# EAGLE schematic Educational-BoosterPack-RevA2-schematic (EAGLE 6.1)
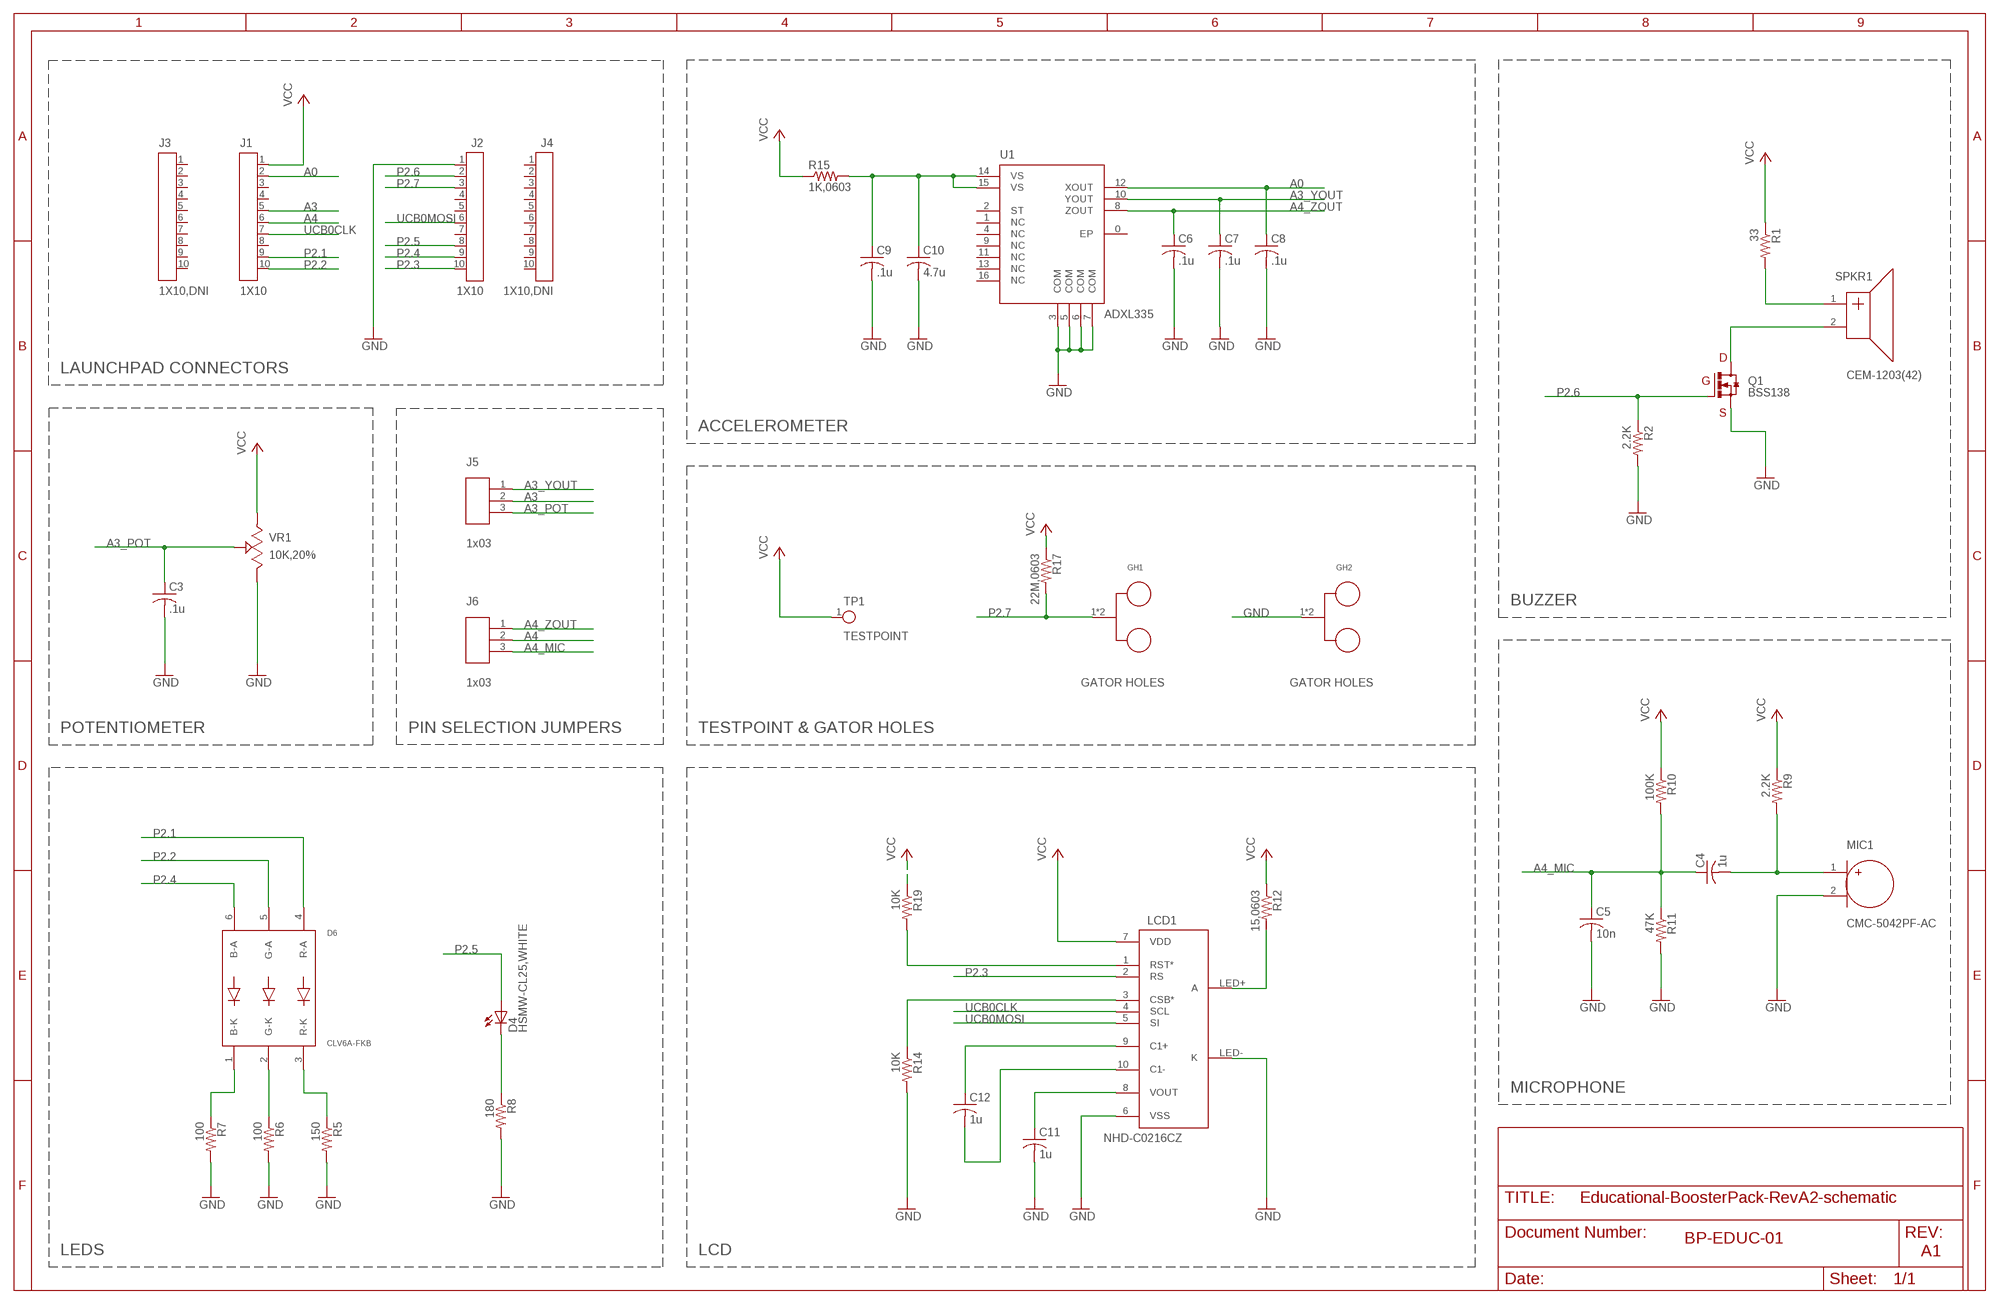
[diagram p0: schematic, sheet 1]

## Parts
C3  .1u  C-USC0402  [C0402]
C4  1u  C-USC0402  [C0402]
C5  10n  C-USC0402  [C0402]
C6  .1u  C-USC0402  [C0402]
C7  .1u  C-USC0402  [C0402]
C8  .1u  C-USC0402  [C0402]
C9  .1u  C-USC0402  [C0402]
C10  4.7u  C-USC0603  [C0603]
C11  1u  C-USC0402  [C0402]
C12  1u  C-USC0402  [C0402]
D4  HSMW-CL25,WHITE  LEDCHIPLED_0603  [CHIPLED_0603]
D6  CLV6A-FKB  [TRICOLOR-LED6]
GH1  MAKEYMAKEY  [MAKEYMAKEY]
GH2  MAKEYMAKEY  [MAKEYMAKEY]
J1  1X10  HEADER1X10  [1X10]
J2  1X10  HEADER1X10  [1X10]
J3  1X10,DNI  HEADER1X10  [1X10]
J4  1X10,DNI  HEADER1X10  [1X10]
J5  1x03  HEADER1X03  [1X03]
J6  1x03  HEADER1X03  [1X03]
LCD1  NHD-C0216CZ  [GENERIC-LCD10-2]
MIC1  CMC-5042PF-AC  [GENERIC-2PADS2]
Q1  BSS138  [SOT23-3]
R1  33  R-US_R0402  [R0402]
R2  2.2K  R-US_R0402  [R0402]
R5  150  R-US_R0402  [R0402]
R6  100  R-US_R0402  [R0402]
R7  100  R-US_R0402  [R0402]
R8  180  R-US_R0402  [R0402]
R9  2.2K  R-US_R0402  [R0402]
R10  100K  R-US_R0402  [R0402]
R11  47K  R-US_R0402  [R0402]
R12  15,0603  R-US_R0603  [R0603]
R14  10K  R-US_R0402  [R0402]
R15  1K,0603  R-US_R0603  [R0603]
R17  22M,0603  R-US_R0603  [R0603]
R19  10K  R-US_R0402  [R0402]
SPKR1  CEM-1203(42)  [GENERIC-2PADS]
TP1  TESTPOINT  [TESTPOINT]
U1  ADXL335  [LFCSP-16]
VR1  10K,20%  3352T  [GENERIC-3HOLES]

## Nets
A0: C8.1 J1.2 U1.12(XOUT)
A3: J1.5 J5.2
A3_POT: C3.1 J5.3 VR1.2
A3_YOUT: C7.1 J5.1 U1.10(YOUT)
A4: J1.6 J6.2
A4_MIC: C4.1 C5.1 J6.3 R10.2 R11.1
A4_ZOUT: C6.1 J6.1 U1.8(ZOUT)
GND: C3.2 C5.2 C6.2 C7.2 C8.2 C9.2 C10.2 C11.2 GH2.1 GH2.2 J2.1 LCD1.6(VSS) LCD1.LED-(K) MIC1.2(MIC_N) Q1.2(S) R2.2 R5.2 R6.2 R7.2 R8.2 R11.2 R14.2 U1.3(COM) U1.5(COM) U1.6(COM) U1.7(COM) VR1.3
N$1: C9.1 C10.1 R15.2 U1.14(VS) U1.15(VS)
N$2: C4.2 MIC1.1(MIC_P) R9.2
N$3: LCD1.LED+(A) R12.2
N$4: D6.2(G-K) R6.1
N$5: R1.2 SPKR1.1(SPKR_P)
N$6: Q1.3(D) SPKR1.2(SPKR_N)
N$7: LCD1.3(CSB*) R14.1
N$8: D6.3(R-K) R5.1
N$9: D6.1(B-K) R7.1
N$10: C11.1 LCD1.8(VOUT)
N$11: C12.2 LCD1.10(C1-)
N$12: C12.1 LCD1.9(C1+)
N$13: LCD1.1(RST*) R19.2
N$16: D4.C R8.1
P2.1: D6.4(R-A) J1.9
P2.2: D6.5(G-A) J1.10
P2.3: J2.10 LCD1.2(RS)
P2.4: D6.6(B-A) J2.9
P2.5: D4.A J2.8
P2.6: J2.2 Q1.1(G) R2.1
P2.7: GH1.1 GH1.2 J2.3 R17.2
UCB0CLK: J1.7 LCD1.4(SCL)
UCB0MOSI: J2.6 LCD1.5(SI)
VCC: J1.1 LCD1.7(VDD) R1.1 R9.1 R10.1 R12.1 R15.1 R17.1 R19.1 TP1.1 VR1.1
Unconnected: J1.3 J1.4 J1.8 J2.4 J2.5 J2.7 J3.1 J3.2 J3.3 J3.4 J3.5 J3.6 J3.7 J3.8 J3.9 J3.10 J4.1 J4.2 J4.3 J4.4 J4.5 J4.6 J4.7 J4.8 J4.9 J4.10 U1.0(EP) U1.1(NC) U1.2(ST) U1.4(NC) U1.9(NC) U1.11(NC) U1.13(NC) U1.16(NC)

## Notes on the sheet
- LAUNCHPAD CONNECTORS
- ACCELEROMETER
- BUZZER
- GATOR HOLES | GATOR HOLES
- POTENTIOMETER | PIN SELECTION JUMPERS | TESTPOINT & GATOR HOLES
- MICROPHONE
- BP-EDUC-01
- LEDS | LCD | A1

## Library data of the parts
C3-C12 = resistor:C-US: CAPACITOR, American symbol
D4 = led:LED: LED
D6 = CCo-Boost:CLV6A-FKB
GH1 GH2 = CCo-Boost:MAKEYMAKEY
J1-J4 = CCo-Boost:HEADER1X10
J5 J6 = CCo-Boost:HEADER1X03
LCD1 = CCo-Boost:NHD-C0216CZ
MIC1 = CCo-Boost:CMC-5042PF-AC
Q1 = CCo-Boost:BSS138: BSS138 N-Channel Logic Level Enhancement Mode Field Effect Transistor
R1 R2 R5-R12 R14 R15 R17 R19 = resistor:R-US_: RESISTOR, American symbol
SPKR1 = CCo-Boost:CEM-1203(42)
TP1 = CCo-Boost:TESTPOINT
U1 = CCo-Boost:ADXL335: ADXL335 A small, thin, low power, complete 3-axis accelerometer. The ADXL335 is available in a small, low profile, 4mm x 4mm x 1.45mm, 16-lead, plastic lead frame chip scale package (LFCSP_LQ)
VR1 = CCo-Boost:3352T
